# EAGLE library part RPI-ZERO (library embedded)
Raspberry Pi Zero W BCM 2835 SOC @ 1GHz 1GHz 512MB of RAM On-board Wireless LAN - 2.4 GHz 802.11 b/g/n (BCM43438) On-board Bluetooth 4.1 + HS Low-energy (BLE) (BCM43438) micro-SD mini-HDMI micro-B USB for data micro-B USB for power CSI camera connector (needs adaptor cable) Unpopulated 40-pin GPIO connector (requires soldering) Compatible with existing pHAT/HAT add-ons Dimensions: 65mm x 30mm x 5mm Source: Raspberry Pi Zero W
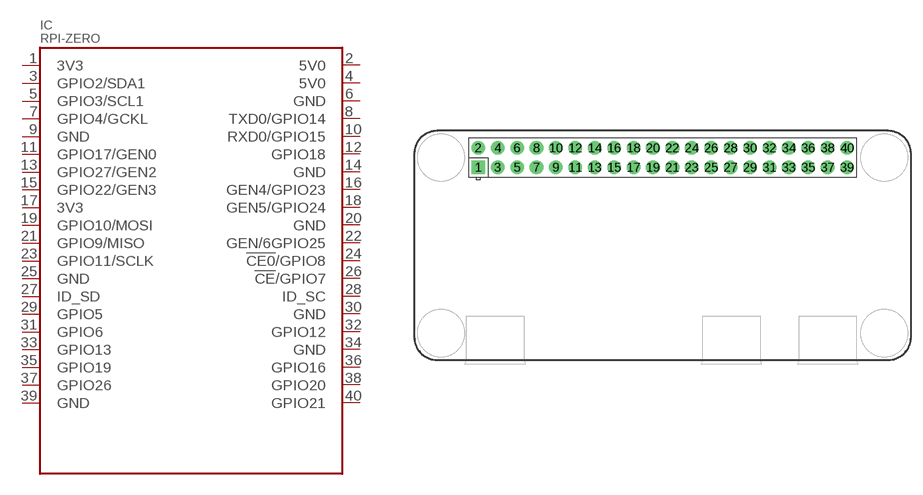
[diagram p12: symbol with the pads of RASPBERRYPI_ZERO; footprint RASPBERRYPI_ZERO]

Designator prefix IC

## RPI-ZERO (DESCR: Raspberry Pi Zero W; MF: Raspberry Pi; UNIT_PRICE: 10.53)  [RASPBERRYPI_ZERO]
1  3V3
2  5V0  sup
3  GPIO2/SDA1
4  5V0  sup
5  GPIO3/SCL1
6  GND  sup
7  GPIO4/GCKL
8  TXD0/GPIO14
9  GND  sup
10  RXD0/GPIO15
11  GPIO17/GEN0
12  GPIO18
13  GPIO27/GEN2
14  GND  sup
15  GPIO22/GEN3
16  GEN4/GPIO23
17  3V3
18  GEN5/GPIO24
19  GPIO10/MOSI
20  GND  sup
21  GPIO9/MISO
22  GEN/6GPIO25
23  GPIO11/SCLK
24  !CE0!/GPIO8
25  GND  sup
26  !CE!/GPIO7
27  ID_SD
28  ID_SC
29  GPIO5
30  GND  sup
31  GPIO6
32  GPIO12
33  GPIO13
34  GND  sup
35  GPIO19
36  GPIO16
37  GPIO26
38  GPIO20
39  GND  sup
40  GPIO21

## Footprint RASPBERRYPI_ZERO (pad centres in mm)
Raspberry Pi board model B+, full outline with position of big connectors & drill holes
drill 1 pad 1.778 square: 1 8.37,25.23
drill 1 pad 1.778: 2 8.37,27.77; 3 10.91,25.23; 4 10.91,27.77; 5 13.45,25.23; 6 13.45,27.77; 7 15.99,25.23; 8 15.99,27.77; 9 18.53,25.23; 10 18.53,27.77; 11 21.07,25.23; 12 21.07,27.77; 13 23.61,25.23; 14 23.61,27.77; 15 26.15,25.23; 16 26.15,27.77; 17 28.69,25.23; 18 28.69,27.77; 19 31.23,25.23; 20 31.23,27.77; 21 33.77,25.23; 22 33.77,27.77; 23 36.31,25.23; 24 36.31,27.77; 25 38.85,25.23; 26 38.85,27.77; 27 41.39,25.23; 28 41.39,27.77; 29 43.93,25.23; 30 43.93,27.77; 31 46.47,25.23; 32 46.47,27.77; 33 49.01,25.23; 34 49.01,27.77; 35 51.55,25.23; 36 51.55,27.77; 37 54.09,25.23; 38 54.09,27.77; 39 56.63,25.23; 40 56.63,27.77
